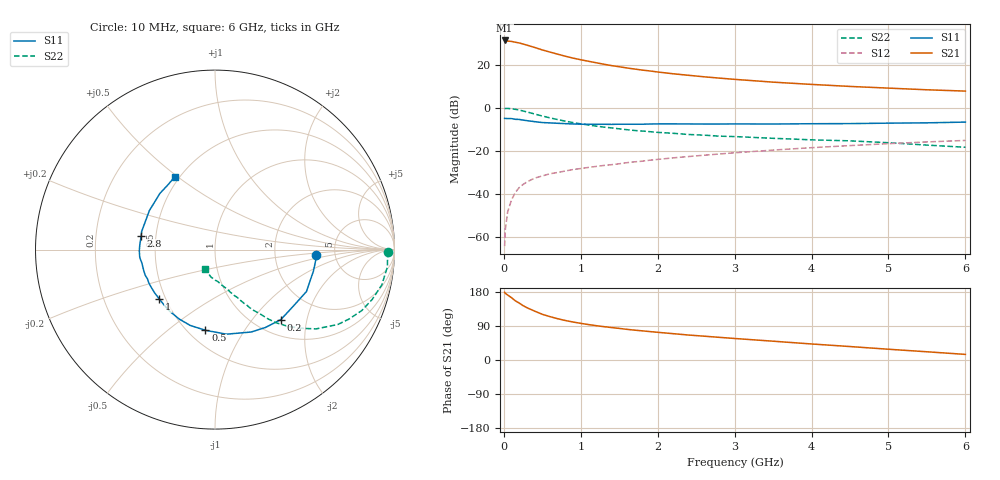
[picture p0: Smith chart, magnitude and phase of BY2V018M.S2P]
! SIEMENS Small Signal Semiconductors
! BFY420
! Si NPN RF SIEGET Grounded Emitter Transistor in MICRO-X
! VCE = 2 V  IC = 18 mA
! Common Emitter S-Parameters:  October  1996
# GHz  S  MA  R  50
!  f  S11  S21  S12  S22
! GHz  MAG  ANG  MAG  ANG  MAG  ANG  MAG  ANG
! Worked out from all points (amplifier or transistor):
!   36 points, 10 MHz to 6 GHz, reference 50 ohm
!   highest |S21| = 31.3 dB at 10 MHz (marker M1)
!   |S21| within 3 dB of that: start of sweep to 376.5 MHz
!   unconditionally stable (mu >= 1): start of sweep to 10.37 MHz; 2.041 GHz to end of sweep
!   at 250 MHz: K = 0.27, MSG = 32.7 dB, |S12| = -35.7 dB
!   at 1.4 GHz: K = 0.90, MSG = 23.1 dB, |S12| = -26.5 dB
!   at 6 GHz: K = 1.08, MAG = 9.8 dB, |S12| = -15.2 dB
!   S11 on the Smith chart (normalised r, x): 10 MHz: 3.58, -0.29; 200 MHz: 1.29, -1.41; 500 MHz: 0.61, -0.69; 1 GHz: 0.46, -0.31; 2.8 GHz: 0.41, +0.08; 6 GHz: 0.47, +0.49
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0.01  0.5655 -2.8  36.91 178.7  0.0006 93.5  0.9634 -0.7
0.02  0.5652 -5.1  36.78 175.8  0.0015 101.4  0.9621 -1.8
0.05  0.5614 -12.2  35.7 171.4  0.0038 86.4  0.9653 -5.7
0.1  0.5605 -24.6  35.05 164.4  0.0072 81.6  0.9498 -12.0
0.15  0.5388 -35.3  33.54 156.2  0.0107 74.7  0.9187 -17.6
0.2  0.5354 -46.7  32.25 150.2  0.0139 72.3  0.8851 -22.6
0.25  0.5171 -57.0  30.48 143.5  0.0164 68.1  0.841 -27.4
0.3  0.5015 -66.3  28.72 138.0  0.0188 66.8  0.8011 -31.4
0.4  0.4755 -82.3  25.38 129.0  0.023 62.1  0.7158 -38.1
0.5  0.4527 -96.8  22.22 120.6  0.0259 59.1  0.6426 -43.0
0.6  0.4444 -108.2  19.8 114.4  0.0291 57.4  0.5821 -46.9
0.7  0.4352 -117.1  17.69 108.9  0.0312 56.4  0.5315 -50.1
0.8  0.4269 -125.7  15.84 104.2  0.0338 54.9  0.4877 -52.5
1  0.4148 -138.2  13.11 96.7  0.0385 55.4  0.423 -55.9
1.1  0.414 -144.2  12.1 93.5  0.0409 55.7  0.3971 -57.9
1.6  0.414 -163.6  8.444 80.9  0.0527 55.1  0.3088 -64.0
2.2  0.4218 -179.0  6.189 69.5  0.0682 53.9  0.2546 -69.9
2.8  0.4182 169.5  4.907 59.8  0.0838 51.2  0.2185 -75.1
3.5  0.4186 157.5  3.951 49.6  0.1035 47.1  0.1946 -80.8
4.5  0.4282 141.9  3.139 35.5  0.1317 39.2  0.1698 -90.0
5.5  0.446 126.0  2.623 21.7  0.1603 30.1  0.1352 -106.3
6  0.4641 118.7  2.446 14.8  0.1737 25.3  0.1205 -118.5
